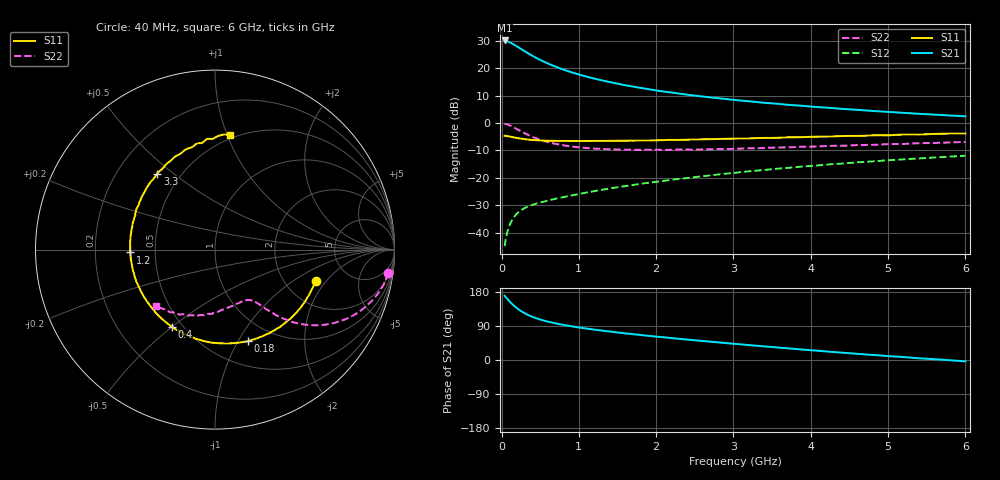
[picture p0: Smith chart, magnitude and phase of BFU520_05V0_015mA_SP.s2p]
! Filename:  P:\Prog\Test\Noise\ATS_data\Testdata_Net\03 Spar\BFU520_APG2013_37_A05_05p0V_015mA_SP_CM01_D.s2p
! Date/Time: Fri 26/Apr/2013 13:00:08
! BFU520_APG2013_37_A05_05p0V_1to20mA_SP_CM01_Bias7_R.s2p
! MDIF S-parameter v. bias file
! BFU520_APG2013_37_A05_05p0V_1to20mA_SP_CM01
! Date/time Tue Apr 23 15:26:19 2013
! VAR V_out= 5.0010
! VAR I_out= 14.9950
! VAR V_in= 0.8432
! VAR I_in= 0.1736
! Device data file deembeded for feedlines and parallel
! Original file: \03 Spar\BFU520_APG2013_37_A05_05p0V_015mA_SP_CM01_R.s2p
! Feed-files: PR047V01_250413_Feed1.s2p, PR047V01_250413_Feed2.s2p
! Parallel-file: PR047V01_250413_Par.s2p
# MHz S MA R 50
!  Freq-MHz  S11-mag  S11-arg  S21-mag  S21-arg  S12-mag  S12-arg  S22-mag  S22-arg
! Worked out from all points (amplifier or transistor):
!   98 points, 40 MHz to 6 GHz, reference 50 ohm
!   highest |S21| = 30.1 dB at 40 MHz (marker M1)
!   |S21| within 3 dB of that: start of sweep to 246.7 MHz
!   unconditionally stable (mu >= 1): 1.477 GHz to 3.501 GHz
!   at 300 MHz: K = 0.40, MSG = 28.6 dB, |S12| = -31.0 dB
!   at 1.6 GHz: K = 1.02, MAG = 17.5 dB, |S12| = -23.0 dB
!   at 6 GHz: K = 0.83, MSG = 7.2 dB, |S12| = -11.9 dB
!   S11 on the Smith chart (normalised r, x): 40 MHz: 2.92, -1.56; 180 MHz: 0.76, -1.10; 400 MHz: 0.44, -0.50; 1.2 GHz: 0.36, -0.01; 3.3 GHz: 0.37, +0.44; 6 GHz: 0.47, +1.02
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40  0.5868 -17.4  32.02 169.6  0.005708 82.9  0.9742 -7.7
50  0.5841 -21.7  31.94 166.6  0.006997 80.8  0.9678 -9.6
80  0.5764 -34.1  30.68 160.0  0.01088 76.2  0.94 -15.2
120  0.5629 -49.8  28.97 151.2  0.01543 70.5  0.8893 -21.7
140  0.5555 -57.0  27.97 147.2  0.01744 67.9  0.8617 -24.7
180  0.5425 -70.3  25.89 140.1  0.02098 63.5  0.8044 -29.7
220  0.5284 -82.1  23.97 133.6  0.02384 60.2  0.7491 -33.8
280  0.5134 -96.9  21.16 125.7  0.02726 56.6  0.6742 -38.6
340  0.5003 -109.1  18.81 119.2  0.03 54.3  0.6121 -42.0
400  0.4922 -119.2  16.81 113.9  0.03227 53.0  0.5606 -44.3
500  0.4828 -132.6  14.15 106.9  0.03571 52.0  0.4964 -47.1
650  0.4753 -147.3  11.37 98.8  0.04026 52.2  0.4325 -49.5
800  0.4727 -157.9  9.441 92.7  0.04477 53.2  0.3931 -51.1
1050  0.4712 -171.7  7.341 84.4  0.05253 55.1  0.3562 -53.6
1200  0.4725 -178.1  6.465 80.1  0.05738 56.0  0.3432 -55.2
1600  0.4769 167.8  4.896 70.3  0.07097 57.5  0.3276 -60.4
2050  0.487 155.9  3.835 60.9  0.08656 57.9  0.325 -67.5
3100  0.5221 131.3  2.568 41.2  0.1275 55.6  0.3429 -85.6
3300  0.532 127.2  2.417 37.6  0.1359 54.7  0.3477 -89.1
4100  0.5654 112.1  1.95 24.3  0.1697 50.1  0.3745 -103.3
5200  0.6192 94.0  1.535 7.8  0.2183 42.2  0.4159 -122.6
6000  0.6448 82.7  1.327 -3.5  0.2533 35.4  0.4535 -136.3
